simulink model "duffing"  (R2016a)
settings: Solver=ode23tb  StartTime=0.0  StopTime=100  RelTol=1e-5
libraries: simulink x1

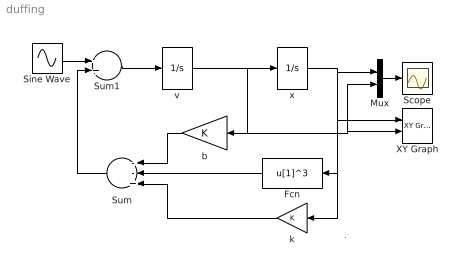
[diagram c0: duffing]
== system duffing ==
  note: .
  Fcn : Fcn  Expr=u[1]^3
  Mux : Mux  Inputs=2
  Scope : Scope
  Sine Wave : Sin  Phase=pi/2  SampleTime=0
  Sum : Sum  Inputs=--+
  Sum1 : Sum
  XY Graph : simulink/Sinks/XY Graph  xmin=-2  xmax=2  ymin=-2  ymax=2  st=-1
  b : Gain
  k : Gain
  v : Integrator
  x : Integrator
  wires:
  v/1 -> b/1, XY Graph/2, Mux/2, x/1
  x/1 -> k/1, Fcn/1, XY Graph/1, Mux/1
  b/1 -> Sum/1
  Sum1/1 -> v/1
  Sum/1 -> Sum1/2
  Fcn/1 -> Sum/2
  k/1 -> Sum/3
  Sine Wave/1 -> Sum1/1
  Mux/1 -> Scope/1
